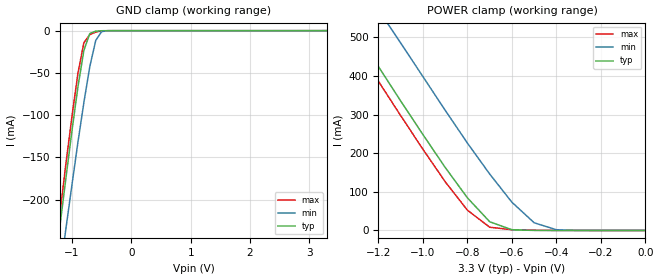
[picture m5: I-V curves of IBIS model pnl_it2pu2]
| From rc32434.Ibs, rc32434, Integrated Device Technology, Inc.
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[Model]   pnl_it2pu2
Model_type   Input
Polarity   Non-Inverting
Enable   Active-High
Vinl =  0.800V
Vinh =  2.000V
C_comp   0.40pF   0.30pF   0.50pF
[Temperature Range]   25.00   0.12k   0.000
[Voltage Range]   3.30V   3.00V   3.60V
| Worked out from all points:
|   GND clamp passes 1 mA (typ) near -0.62 V on its own axis
|   POWER clamp passes 1 mA (typ) near -0.55 V on its own axis
[GND_clamp]
| voltage   I(typ)   I(min)   I(max)
-3.3V     -1.469A    -1.42A     -1.487A
-1.3V     -286mA     -337mA     -272mA
-1.2V     -229mA     -285mA     -214mA
-1.1V     -173mA     -233mA     -156mA
-1V       -118mA     -182mA     -101mA
-900mV    -66.54mA   -132mA     -50.36mA
-800mV    -23.33mA   -85.12mA   -14.25mA
-700mV    -3.351mA   -42.49mA   -4.631mA
-600mV    -559uA     -11.57mA   -1.686mA
-500mV    -80.05uA   -1.102mA   -334uA
-300mV    -14.63uA   -11.9uA    -22.24uA
3.3V      277pA      104uA      692nA
[POWER_clamp]
| voltage   I(typ)   I(min)   I(max)
-3.3V     2.292A     2.4A       2.265A
-1.4V     601mA      745mA      565mA
-1.3V     513mA      658mA      475mA
-1.2V     424mA      571mA      386mA
-1.1V     335mA      485mA      297mA
-900mV    163mA      311mA      126mA
-800mV    84.3mA     226mA      52.35mA
-700mV    22.57mA    146mA      8.389mA
-600mV    1.773mA    72.93mA    1.942mA
-500mV    197uA      19.88mA    605uA
-400mV    23.11uA    1.826mA    89.72uA
0V        277pA      1.066nA    351pA
